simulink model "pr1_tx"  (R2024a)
settings: Solver=FixedStepDiscrete  StartTime=0  StopTime=0.5  RelTol=1e-3
StartFcn:
  | assert(c.AllowTransmit, ...
  |     'Set the assigned TX slot first');
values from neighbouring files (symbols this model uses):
  c = dpo_config(1)    [check_project.m]    (also in main_practice1.m)
  w = w.*exp(2j*pi*c.Shift*n/c.Fs)    [dpo_waveform.m]
undefined symbols (not defined in the file or in its folder): Fs, ip, repmat
libraries: ad936xlib x1

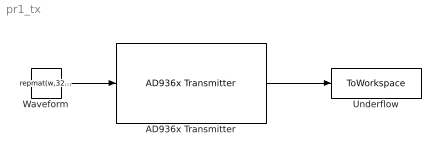
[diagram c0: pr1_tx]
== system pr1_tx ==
  AD936x Transmitter : ad936xlib/AD936x Transmitter  IPAddress=169.254.0.52  uri=ip:10.0.0.200  CenterFrequencySource=Dialog  CenterFrequency=c.RF  GainSource=Dialog  Gain=c.TxGain  ChannelMapping=1  BasebandSampleRate=c.Fs  UnderflowOutputPort=on  ShowAdvancedProperties=off  UseCustomFilter=off  filtPathRates=[737280000 11520000 3840000 1920000 960000 240000]  filtCoefficients="[-192 82 85 -215 228 -102 -110 290 -318 145 160 -426 471 -215 -238 633 -697 318 349 -923 1009 -457 -498 1309 -1423 640 693 -1812 1959 -876 -945 2458 -2647 1180 1268 -3290 3534 -1572 -1688 4375 -4698 2091 2247 -5836 6284 -2807 -3031 7918 -8588 3870 4225 -11182 12324 -5662 -6330 17255 -19735 9507 11312 -33568 43355 -25227 -42139 305542 305542 -42139 -25227 43355 -33568 11312 9507 -19735 17255 -6330 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"  filtCoefficientSize=128  filtDecimInterpFactor=4  filtGain=-12  filtRFBandwidth=18000000  filterConfigStruct=struct()  BypassUserLogic=off  DataSourceSelect=Input Port  DDSTone1Freq=5000  DDSTone2Freq=10000  DDSTone1Scale=0.5  DDSTone2Scale=0.25  DataTimeout=Inf  ENSMPinControlMode=None  BISTLoopbackMode=Disabled  BISTToneInject=Disabled  BISTSignalGen=PRBS  BISTToneFreq=Fs/32  BISTToneLevel=0
  Underflow : ToWorkspace  VariableName=txUnderflow  SampleTime=-1
  Waveform : Constant  Value=repmat(w,32,1)  VectorParams1D=off  SampleTime=32*numel(w)/c.Fs
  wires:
  Waveform/1 -> AD936x Transmitter/1
  AD936x Transmitter/1 -> Underflow/1
